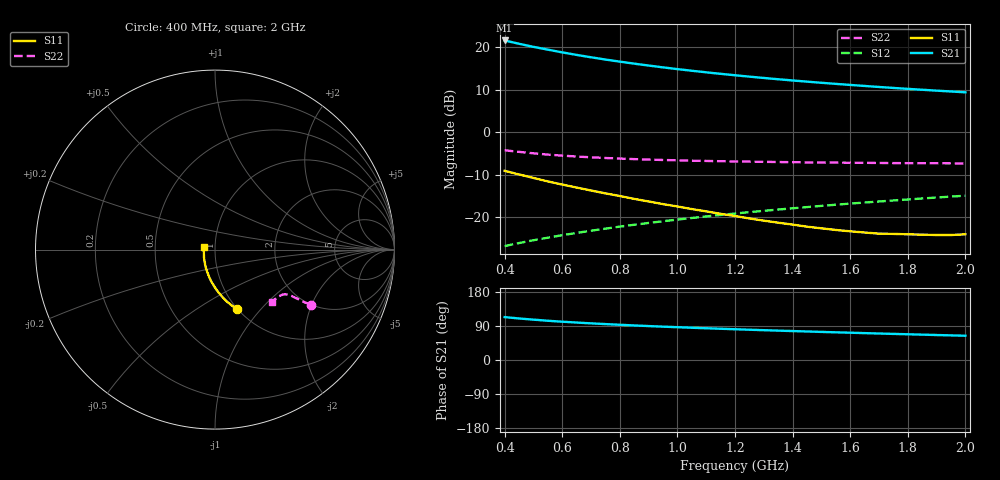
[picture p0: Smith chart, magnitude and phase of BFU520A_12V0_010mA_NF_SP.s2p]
! Filename:  P:\Prog\Test\Noise\ATS_data\Testdata_Net\06 Compressed Noise after Statistics\BFU520A_APG2013_30_A05_12p0V_010mA_NF_CM01_D.sf
! Date/Time: Wed 24/Apr/2013 20:06:21
! BFU520A_APG2013_30_A05_12p0V_1to20mA_NF_CM01_Bias6_R.sf
! Noise Parameter Data File
! BFU520A_APG2013_30_A05_12p0V_1to20mA_NF_CM01
! Date/time: Thu Apr 11 10:46:45 2013
! VAR V_out= 12.001000
! VAR I_out= 9.995000
! VAR V_in= 0.813900
! VAR I_in= 0.099910
! Device data file deembeded for feedlines and parallel
! Original file: \06 Compressed Noise after Statistics\BFU520A_APG2013_30_A05_12p0V_010mA_NF_CM01_R.sf
! Feed-files: PR017V01_150413_Feed1.s2p, PR017V01_150413_Feed2.s2p
! Parallel-file: PR017V01_150413_Par.s2p
# MHz S MA R 50
!  Freq-MHz  S11-mag  S11-arg  S21-mag  S21-arg  S12-mag  S12-arg  S22-mag  S22-arg
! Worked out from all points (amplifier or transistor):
!   37 points, 400 MHz to 2 GHz, reference 50 ohm
!   highest |S21| = 21.5 dB at 400 MHz (marker M1)
!   |S21| within 3 dB of that: start of sweep to 616.9 MHz
!   unconditionally stable (mu >= 1): 1.357 GHz to end of sweep
!   at 500 MHz: K = 0.81, MSG = 22.7 dB, |S12| = -25.4 dB
!   at 1.1 GHz: K = 0.98, MSG = 16.9 dB, |S12| = -19.8 dB
!   at 2 GHz: K = 1.01, MAG = 11.7 dB, |S12| = -14.9 dB
!   lowest NFmin = 0.85 dB at 420 MHz
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400  0.352 -69.7  11.94 113.3  0.04588 68.6  0.6141 -29.9
420  0.3387 -71.5  11.52 111.7  0.04753 68.7  0.6027 -30.1
440  0.325 -73.3  11.12 110.3  0.04913 68.7  0.5924 -30.3
460  0.3133 -74.7  10.74 109.0  0.0507 68.8  0.5829 -30.4
480  0.3019 -76.4  10.39 107.7  0.05227 68.8  0.5732 -30.5
500  0.2904 -77.9  10.05 106.5  0.05386 68.9  0.5652 -30.6
550  0.2641 -81.6  9.321 103.6  0.05772 69.2  0.5453 -30.8
600  0.2428 -84.7  8.653 101.1  0.06173 69.4  0.5308 -30.8
650  0.224 -87.8  8.083 98.8  0.06567 69.7  0.518 -31.0
700  0.2067 -90.8  7.579 96.7  0.0697 69.9  0.5072 -31.1
750  0.1913 -93.7  7.13 94.8  0.07374 70.2  0.4979 -31.2
800  0.1782 -96.8  6.735 93.0  0.07779 70.3  0.49 -31.4
850  0.1648 -99.7  6.38 91.2  0.08186 70.4  0.4829 -31.6
950  0.1431 -105.5  5.769 88.0  0.09002 70.7  0.4717 -32.0
1050  0.1251 -111.4  5.265 85.1  0.09829 70.8  0.4629 -32.5
1150  0.11 -118.3  4.846 82.5  0.1067 70.7  0.456 -33.2
1200  0.1037 -121.5  4.662 81.2  0.1109 70.7  0.4532 -33.6
1350  0.08652 -132.6  4.184 77.5  0.1235 70.5  0.4464 -34.9
1500  0.07438 -145.8  3.803 74.1  0.1363 70.1  0.4404 -36.4
1650  0.06639 -159.6  3.49 70.9  0.1493 69.5  0.4369 -38.1
1750  0.06394 -170.1  3.308 68.9  0.1579 69.2  0.4338 -39.3
2000  0.06325 166.4  2.94 64.0  0.1797 68.0  0.4297 -42.6
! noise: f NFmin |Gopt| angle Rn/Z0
400  0.9108  0.01969  -71.57  0.1183
460  0.8762  0.00449  -157.2  0.1091
600  0.9955  0.02667  -51.5  0.1382
800  0.9315  0.0319  151.4  0.1048
1000  0.9551  0.03769  178.9  0.1026
1200  1.013  0.0385  -173  0.1077
1400  1.018  0.06576  179.2  0.1014
1600  1.03  0.08993  -139.8  0.103
1800  0.9997  0.1303  -151.2  0.0907
2000  1.038  0.1427  -138.7  0.0977
